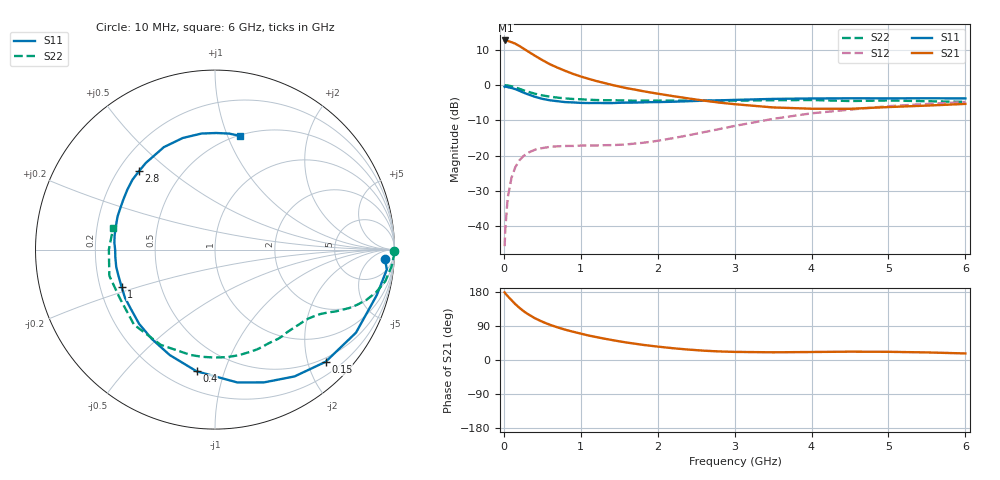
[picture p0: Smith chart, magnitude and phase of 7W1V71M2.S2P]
! Infineon Technologies  Discrete & RF Semiconductors
! BFS17W
! Si NPN RF Bipolar Junction Transistor in SOT323
! VCE = 1.75 V  IC = 1.2 mA
! Common Emitter S-Parameters:  August  1999
# GHz  S  MA  R  50
!  f  S11  S21  S12  S22
! GHz  MAG  ANG  MAG  ANG  MAG  ANG  MAG  ANG
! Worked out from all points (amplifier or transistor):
!   36 points, 10 MHz to 6 GHz, reference 50 ohm
!   highest |S21| = 12.7 dB at 20 MHz (marker M1)
!   |S21| within 3 dB of that: start of sweep to 306.1 MHz
!   unconditionally stable (mu >= 1): 945.4 MHz to end of sweep
!   at 250 MHz: K = 0.29, MSG = 15.3 dB, |S12| = -20.2 dB
!   at 1.4 GHz: K = 1.33, MAG = 5.1 dB, |S12| = -17.0 dB
!   at 6 GHz: K = 1.12, MAG = -2.4 dB, |S12| = -4.8 dB
!   S11 on the Smith chart (normalised r, x): 10 MHz: 19, -19; 150 MHz: 0.43, -2.32; 400 MHz: 0.32, -0.81; 1 GHz: 0.29, -0.18; 2.8 GHz: 0.28, +0.40; 6 GHz: 0.51, +1.11
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0.01  0.9479 -3.0  4.278 178.5  0.0052 87.7  0.9993 -0.6
0.02  0.9638 -6.6  4.305 175.5  0.0093 84.2  0.9965 -2.2
0.05  0.9364 -15.7  4.235 168.5  0.0252 81.8  0.9882 -5.4
0.1  0.9117 -30.5  4.07 157.8  0.0488 72.6  0.9652 -10.5
0.15  0.8779 -45.4  3.868 147.2  0.069 64.2  0.9287 -14.8
0.2  0.8341 -57.9  3.604 138.2  0.0853 58.2  0.8898 -18.3
0.25  0.7887 -69.7  3.333 130.0  0.0973 51.6  0.8498 -21.2
0.3  0.7509 -80.4  3.077 122.8  0.108 47.5  0.816 -23.5
0.4  0.6857 -98.6  2.63 110.6  0.1209 40.5  0.7574 -27.0
0.5  0.6394 -113.2  2.268 101.0  0.128 35.8  0.7156 -29.4
0.6  0.6096 -125.3  1.978 92.9  0.1334 32.9  0.6863 -31.6
0.8  0.5742 -144.3  1.592 79.9  0.1371 30.0  0.6484 -36.2
1  0.5607 -158.1  1.327 69.6  0.1389 30.1  0.6301 -40.7
1.1  0.5573 -164.7  1.231 64.7  0.1392 30.4  0.6215 -43.6
1.6  0.5651 171.6  0.905 46.0  0.1446 38.5  0.6037 -57.9
2.2  0.5818 151.4  0.699 31.0  0.1772 51.0  0.6033 -76.9
2.8  0.6086 134.0  0.566 22.6  0.238 56.7  0.6017 -96.8
3.5  0.6381 116.5  0.483 20.3  0.3326 54.7  0.6108 -119.7
4  0.6472 106.1  0.463 21.1  0.3987 49.3  0.6153 -137.2
4.5  0.6511 96.6  0.462 22.0  0.4495 43.0  0.5955 -152.9
5.5  0.6512 83.0  0.513 20.0  0.5412 31.0  0.5913 -180.0
6  0.6486 77.8  0.542 17.3  0.577 25.3  0.58 168.0
